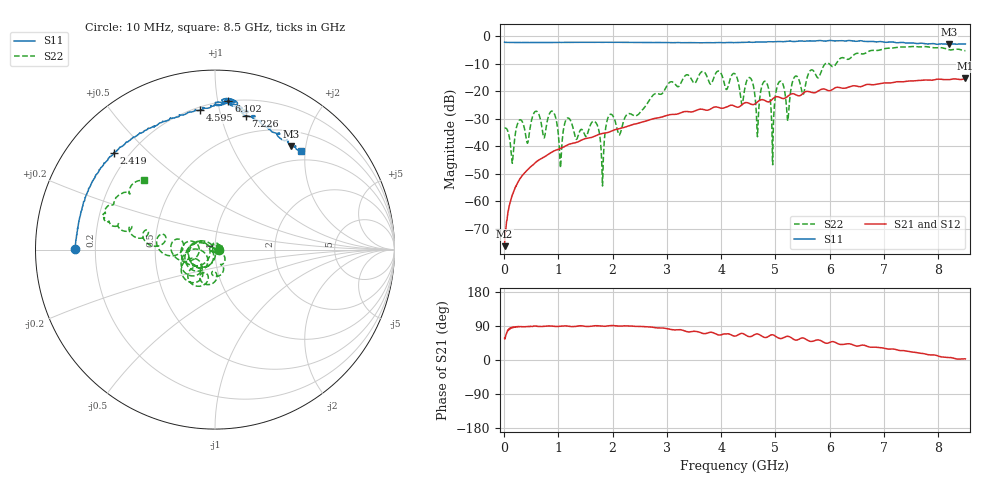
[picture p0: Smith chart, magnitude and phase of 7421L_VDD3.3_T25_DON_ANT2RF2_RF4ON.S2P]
!Agilent Technologies,E5071C,MY46417908,A.11.23
!Date: Thu Feb 25 16:17:24 2021
!Data & Calibration Information:
!Freq	S11:SOLT2(ON)	S21:SOLT2(ON)	S12:SOLT2(ON)	S22:SOLT2(ON)
!PortZ  Port1:50+j0  Port2:50+j0
!Above PortZ is port z conversion or system Z0 setting when saving the data.
!When reading, reference impedance value at option line is always used.
# Hz S dB R 50
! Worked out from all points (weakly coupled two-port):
!   1601 points, 10 MHz to 8.5 GHz, reference 50 ohm
!   highest |S21| = -15.31 dB at 8.5 GHz (marker M1); lowest = -76.4 dB at 10 MHz (marker M2)
!   lowest |S11| = -2.9 dB at 8.192 GHz (marker M3), VSWR 6.03, Z = 36.9 + j87 ohm
!   |S11| at or under -10 dB: nowhere
!   |S22| runs from -54.5 to -3.7 dB; largest |S21 - S12| = 0.0024
!   S11 on the Smith chart (normalised r, x): 10 MHz: 0.12, +0.00; 2.419 GHz: 0.14, +0.39; 4.595 GHz: 0.22, +0.88; 6.102 GHz: 0.20, +1.07; 7.226 GHz: 0.33, +1.20; 8.5 GHz: 0.82, +1.92
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1e7  -2.13 179.7  -76.38 57.4  -75.33 69.6  -33.34 -2.9
1.532688e8  -2.19 176.7  -57.55 85.6  -57.68 85.1  -46.20 17.2
3.28375e8  -2.22 173.1  -50.87 87.7  -50.84 87.5  -30.80 14.0
1.426769e9  -2.16 153.3  -37.71 90.3  -37.73 90.1  -33.83 43.6
1.686775e9  -2.13 148.5  -36.18 90.4  -36.17 90.3  -31.26 94.4
1.808819e9  -2.15 146.8  -35.34 89.2  -35.33 89.1  -52.55 50.5
1.941475e9  -2.13 144.6  -34.76 90.5  -34.76 90.4  -28.61 97.0
2.419038e9  -2.17 136.3  -31.85 88.8  -31.86 88.8  -28.94 -5.5
2.843538e9  -2.20 129.5  -29.65 84.5  -29.65 84.5  -20.90 -68.5
4.255e9  -2.23 102.0  -25.46 63.1  -25.46 63.1  -13.66 -154.8
4.5946e9  -2.14 96.1  -24.82 65.2  -24.80 65.0  -18.01 166.7
4.668888e9  -2.01 94.6  -23.87 68.7  -23.89 68.6  -36.53 -150.8
4.833381e9  -2.01 91.8  -23.65 59.6  -23.63 59.4  -16.75 -175.4
4.950119e9  -1.95 91.4  -22.73 66.4  -22.71 66.4  -46.73 -91.7
5.066856e9  -1.88 90.2  -22.10 57.4  -22.08 57.4  -16.61 -148.8
5.226044e9  -1.74 87.5  -21.81 62.5  -21.81 62.6  -30.77 -175.7
5.671769e9  -1.70 85.9  -20.41 49.1  -20.38 49.3  -12.17 175.3
6.101575e9  -1.62 84.8  -18.69 46.8  -18.70 47.1  -10.44 175.0
7.088538e9  -2.06 76.4  -16.92 28.9  -16.95 28.5  -4.27 165.1
7.2265e9  -2.31 77.1  -16.54 27.2  -16.54 27.2  -4.03 165.7
8.192238e9  -2.91 53.5  -15.76 6.4  -15.79 6.1  -4.82 146.5
8.5e9  -2.75 48.9  -15.31 2.9  -15.37 2.5  -5.19 135.6
